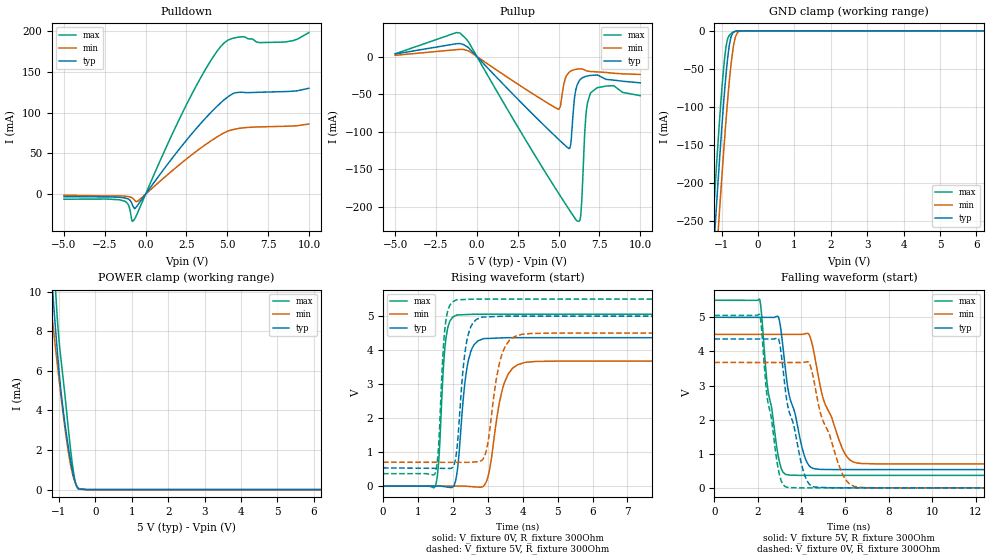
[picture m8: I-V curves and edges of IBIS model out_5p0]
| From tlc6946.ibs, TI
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|   out_5p0 Model
[Model]   out_5p0
Model_type   3-state
Polarity   Non-Inverting
Vmeas = 2.5
Vref = 0
Cref = 2pF
Rref = 100000
|   typ   min   max
C_comp   3.595pF   3.401pF   3.712pF
|  Where Nom  PVT is Nominal Process, 5.0V,   27C
|   Fast PVT is Strong Process,  5.5V,   -40C
|   Slow PVT is Weak Process,   4.5V,   105C
[Voltage Range]   5   4.5   5.5
|Junction Temperature
[Pullup Reference]   5   4.5   5.5
[Pulldown Reference]   0   0   -0
[Power Clamp Reference]   5   4.5   5.5
[GND Clamp Reference]   0   0   0
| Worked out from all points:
|   slope of the pulldown table from 0 to 0.75 V, typ, clamps not added: 36.2 ohm
|   slope of the pullup table from 0 to 0.75 V, typ, clamps not added: 43.6 ohm
|   GND clamp passes 1 mA (typ) near -0.65 V on its own axis
|   POWER clamp passes 1 mA (typ) near -0.64 V on its own axis
|   falling waveform, V_fixture 5V, R_fixture 300Ohm: 20-80 % time 786ps typ, 1.05ns min, 578ps max; typ from 5 V to 0.536 V
|   rising waveform, V_fixture 0V, R_fixture 300Ohm: 20-80 % time 236ps typ, 354ps min, 158ps max; typ from 0 V to 4.37 V
|   rising waveform, V_fixture 5V, R_fixture 300Ohm: 20-80 % time 226ps typ, 335ps min, 154ps max; typ from 0.536 V to 5 V
|   falling waveform, V_fixture 0V, R_fixture 300Ohm: 20-80 % time 787ps typ, 1.05ns min, 579ps max; typ from 4.37 V to 0 V
[Pulldown]
|   Voltage   I(typ)   I(min)   I(max)
-5V       -3.149mA   -1.326mA   -6.216mA
-1.25V    -4.699mA   -2.501mA   -8.846mA
-1.025V   -6.475mA   -3.13mA    -14.67mA
-785mV    -14.36mA   -5.204mA   -33.37mA
-680mV    -17.92mA   -7.341mA   -30.72mA
-485mV    -13.53mA   -8.716mA   -22.68mA
2.485V    65.84mA    42.93mA    109.3mA
4.585V    112mA      72.89mA    181.1mA
5.635V    125mA      80.56mA    192.8mA
6.985V    125.3mA    82.7mA     186.3mA
8.5V      126mA      83.4mA     186.9mA
10V       130.2mA    86.22mA    198.6mA
[GND Clamp]
|   Voltage   I(typ)   I(min)   I(max)
-5V       -3.248A    -3.186A    -3.319A
-1.25V    -313.4mA   -379mA     -262.1mA
-1.145V   -234.4mA   -301mA     -182mA
-1.07V    -180.1mA   -246.8mA   -128mA
-980mV    -118.7mA   -184.2mA   -69.8mA
-905mV    -72.77mA   -135mA     -31.64mA
-845mV    -41.73mA   -98.4mA    -12.92mA
-785mV    -18.48mA   -65.53mA   -5.873mA
-665mV    -1.286mA   -17.75mA   -1.46mA
-560mV    -151.4uA   -2.063mA   -178.7uA
-455mV    -5.842uA   -114.9uA   -4.923uA
10V       0A         0A         0A
[Pullup]
|   Voltage   I(typ)   I(min)   I(max)
-5V       3.376mA    1.643mA    3.652mA
-1.01V    17.19mA    9.523mA    30.8mA
4.99V     -109.8mA   -70.07mA   -181.3mA
5.635V    -122.2mA   -21.14mA   -202.9mA
5.755V    -115.1mA   -19.24mA   -206.8mA
5.95V     -60.36mA   -17.57mA   -213.2mA
6.145V    -37.6mA    -16.71mA   -218.7mA
6.355V    -30mA      -16.36mA   -211.7mA
6.67V     -26.34mA   -18.59mA   -79.49mA
6.94V     -25.16mA   -19.87mA   -49.36mA
8.365V    -31.28mA   -22.17mA   -38.67mA
10V       -34.95mA   -23.81mA   -51.95mA
[POWER Clamp]
|   Voltage   I(typ)   I(min)   I(max)
-5V       116.9mA    79.29mA    328mA
-1.25V    11.92mA    9.77mA     15.91mA
-1.175V   10.04mA    8.486mA    12.95mA
-1.13V    8.948mA    7.726mA    11.29mA
-1.1V     8.237mA    7.224mA    10.26mA
-950mV    5.057mA    4.798mA    6.662mA
-830mV    3.223mA    3.02mA     4.658mA
-725mV    1.934mA    1.697mA    2.762mA
-590mV    612.6uA    537uA      752.5uA
-530mV    239.4uA    239.3uA    233.1uA
-455mV    35.59uA    53.21uA    18.81uA
10V       0A         0A         0A
[Ramp]
R_load = 300
|   typ   min   max
dV/dt_r   2.61959/2.34947e-10   2.20581/3.52341e-10   3.03361/1.57385e-10
dV/dt_f   2.67852/7.84953e-10   2.27892/1.04936e-09   3.08047/5.77132e-10
[Falling Waveform]
V_fixture = 5V
V_fixture_min = 4.5V
V_fixture_max = 5.5V
R_fixture = 300Ohm
C_fixture = 0F
|   Time   V(typ)   V(min)   V(max)
0s        5V         4.5V       5.5V
2.084ns   4.999V     4.499V     5.521V
2.42ns    4.998V     4.499V     3.097V
2.938ns   5.015V     4.499V     924.7mV
3.258ns   3.519V     4.499V     401.7mV
3.453ns   2.67V      4.499V     375mV
4.344ns   654.2mV    4.494V     366.3mV
5.023ns   540.1mV    2.564V     366.2mV
6.417ns   536.4mV    750mV      366.2mV
20ns      535.8mV    701.8mV    365.9mV
[Rising Waveform]
V_fixture = 0V
V_fixture_min = 0V
V_fixture_max = 0V
R_fixture = 300Ohm
C_fixture = 0F
|   Time   V(typ)   V(min)   V(max)
0s        -497.8nV   -149.5nV   -116nV
1.498ns   378.7uV    196.5uV    -8.337mV
1.601ns   404.7uV    210uV      806.3mV
1.8ns     -21.57mV   236.2uV    4.327V
2.114ns   352.4mV    277.4uV    5.032V
2.435ns   3.652V     -8.121mV   5.048V
2.879ns   4.337V     -747.7uV   5.056V
3.47ns    4.362V     3.022V     5.056V
4.065ns   4.366V     3.638V     5.056V
20ns      4.366V     3.676V     5.056V
[Rising Waveform]
V_fixture = 5V
V_fixture_min = 4.5V
V_fixture_max = 5.5V
R_fixture = 300Ohm
C_fixture = 0F
|   Time   V(typ)   V(min)   V(max)
0s        535.8mV    701.8mV    365.9mV
1.491ns   524mV      700.4mV    365.2mV
1.586ns   523.2mV    700.3mV    1.087V
1.788ns   521.6mV    700.1mV    4.766V
2.103ns   985.7mV    699.8mV    5.478V
2.398ns   4.258V     699.6mV    5.492V
2.826ns   4.969V     758.4mV    5.5V
3.398ns   4.996V     3.855V     5.5V
3.961ns   5V         4.461V     5.5V
20ns      5V         4.5V       5.5V
[Falling Waveform]
|Gnd
V_fixture = 0V
V_fixture_min = 0V
V_fixture_max = 0V
R_fixture = 300Ohm
C_fixture = 0F
|   Time   V(typ)   V(min)   V(max)
0s        4.366V     3.676V     5.056V
2.084ns   4.365V     3.676V     5.079V
2.396ns   4.364V     3.675V     2.829V
2.938ns   4.382V     3.675V     548.6mV
3.258ns   2.895V     3.675V     35.99mV
4.344ns   117mV      3.672V     371.5uV
4.886ns   15.67mV    2.156V     358.6uV
5.713ns   602.4uV    670.1mV    339uV
6.417ns   572.7uV    45.85mV    322.2uV
20ns      -500.7nV   -158.6nV   -476.7nV
